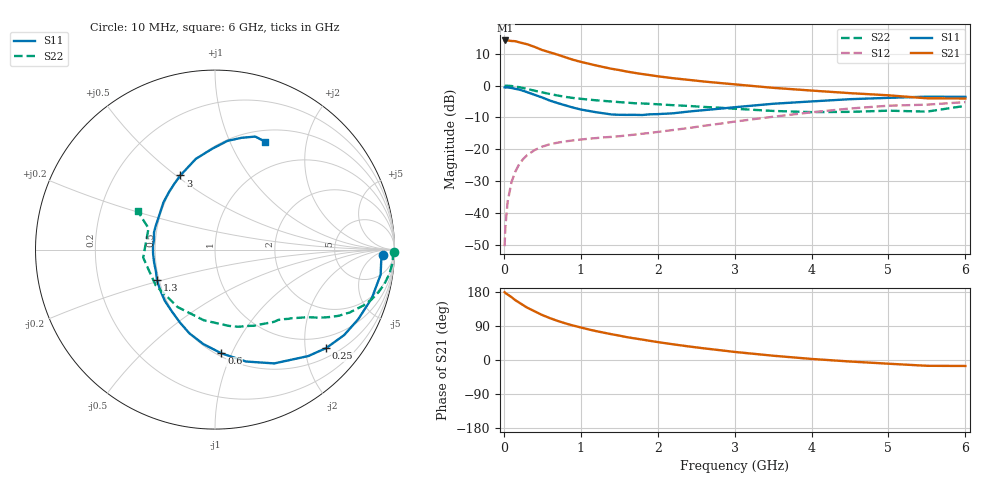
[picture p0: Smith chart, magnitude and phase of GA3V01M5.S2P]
! Infineon Technologies  Discrete & RF Semiconductors
! BF775
! Si NPN RF Bipolar Junction Transistor in SOT23
! VCE = 3 V  IC = 1.5 mA
! Common Emitter S-Parameters:  May  1996
# GHz  S  MA  R  50
!  f  S11  S21  S12  S22
! GHz  MAG  ANG  MAG  ANG  MAG  ANG  MAG  ANG
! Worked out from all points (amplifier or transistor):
!   36 points, 10 MHz to 6 GHz, reference 50 ohm
!   highest |S21| = 14.2 dB at 20 MHz (marker M1)
!   |S21| within 3 dB of that: start of sweep to 498.2 MHz
!   unconditionally stable (mu >= 1): 1.288 GHz to 4.054 GHz; 5.148 GHz to end of sweep
!   at 250 MHz: K = 0.24, MSG = 18.2 dB, |S12| = -23.1 dB
!   at 1.4 GHz: K = 1.07, MAG = 9.1 dB, |S12| = -16.1 dB
!   at 6 GHz: K = 1.01, MAG = -0.2 dB, |S12| = -5.2 dB
!   S11 on the Smith chart (normalised r, x): 10 MHz: 25, -11; 250 MHz: 0.71, -2.46; 600 MHz: 0.53, -0.91; 1.3 GHz: 0.49, -0.19; 3 GHz: 0.50, +0.52; 6 GHz: 0.64, +1.37
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0.01  0.9357 -1.7  5.033 178.9  0.003 89.3  0.9999 -0.7
0.02  0.9281 -3.4  5.101 176.9  0.006 88.4  0.9914 -1.6
0.05  0.9333 -8.6  5.095 172.8  0.0152 84.7  0.9926 -3.9
0.1  0.9146 -17.2  5.002 165.8  0.0306 80.0  0.9821 -7.7
0.15  0.8873 -25.9  4.968 157.7  0.0447 74.8  0.9629 -11.5
0.25  0.8275 -41.5  4.611 144.9  0.0698 65.6  0.915 -17.7
0.3  0.7885 -48.8  4.46 138.5  0.0801 62.3  0.8868 -20.4
0.4  0.7148 -62.5  4.039 128.5  0.0969 55.6  0.8287 -25.0
0.5  0.6471 -74.5  3.604 118.6  0.1097 50.5  0.7793 -28.3
0.6  0.5789 -86.5  3.315 110.4  0.1199 46.9  0.7351 -30.8
0.8  0.4879 -107.0  2.779 96.7  0.1326 42.0  0.6638 -34.7
0.9  0.4503 -115.8  2.538 91.0  0.1376 40.7  0.6373 -36.2
1.1  0.3997 -134.3  2.205 80.8  0.146 39.0  0.6015 -39.2
1.3  0.3656 -152.1  1.944 72.1  0.1534 38.7  0.5727 -41.9
1.6  0.3458 -176.0  1.655 60.3  0.1646 40.0  0.5383 -46.4
2.2  0.3662 147.5  1.302 41.4  0.2001 43.4  0.4911 -57.7
3  0.4561 115.0  1.043 21.3  0.2713 43.0  0.4319 -79.7
3.5  0.5169 101.9  0.92 11.3  0.3233 39.5  0.3989 -98.9
4.5  0.6102 83.4  0.759 -4.0  0.4354 27.8  0.3858 -148.9
5  0.6403 76.6  0.702 -9.8  0.4821 20.1  0.4026 -173.6
5.5  0.6684 70.4  0.63 -15.3  0.5005 11.5  0.3891 162.2
6  0.6633 65.1  0.625 -15.8  0.5495 7.0  0.4801 153.6
